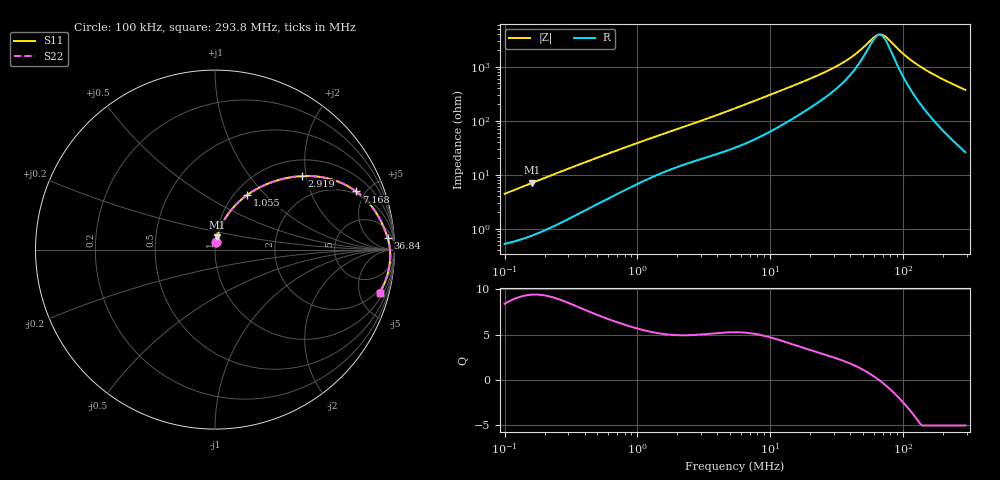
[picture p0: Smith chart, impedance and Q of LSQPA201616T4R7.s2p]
! LSQPA201616T4R7  S-PARAMETER MODEL  ( General Type )
! Model Generated by TAIYO YUDEN Corporation (http://www.ty-top.com)
! Version 2.0
! TAIYO YUDEN Control No. 100810NF25SB-FKC
! Copyright(c) 2007 TAIYO YUDEN CO.,LTD. All Rights Reserved.
! Product Description (link to TY-COMPAS)
! https://ds.yuden.co.jp/TYCOMPAS/or/detail?pn=LSQPA201616T4R7M&u=M
! Products Name : Inductors
! Characteristics :
!  Inductance : 4.7 uH , SRF(min) : 45 MHz , DC Resistance(max) : 0.481 Ohm
!  Rated Current : Saturation :550 mA , Temp Rise : 530 mA (40 degC)
!  Case Size : 2.0 x 1.6 / 0.079 x 0.063 [mm/inch] , Thickness : 1.6 / 0.063 [mm/inch]
!  (Conditions: Temperature = 25 degC , DC Bias Current/Voltage = 0A / 0V)
! External Node Assignments :
!  1  o---GGG---o  2
! GND o---------o GND
! Frequency Range : 0.1MHz  -  293.796821MHz  [ 402 STEP ]
# MHz S RI R 50
! Freq[MHz].  S11 Real  S11 Imag  S21 Real  S21 Imag  S12 Real  S12 Imag  S22 Real  S22 Imag
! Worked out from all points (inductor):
!   401 points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, 100 kHz to 293.8 MHz, reference 50 ohm
!   read as one part in series: L = 6.94 uH near 104.1 kHz
!   highest Q = 9.41 at 161.5 kHz (marker M1), where L = 6.91 uH
!   self-resonance near 65.8 MHz
!   S11 on the Smith chart (normalised r, x): 100 kHz: 1.01, +0.09; 1.055 MHz: 1.14, +0.80; 2.919 MHz: 1.38, +1.90; 7.168 MHz: 1.84, +4.31; 36.84 MHz: 12, +23; 293.8 MHz: 1.52, -7.39
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0.1  0.00706 0.0432  0.9929 -0.0432  0.9929 -0.0432  0.00706 0.0432
0.161467  0.0122 0.0687  0.9878 -0.0687  0.9878 -0.0687  0.0122 0.0687
0.380976  0.0431 0.1493  0.9569 -0.1493  0.9569 -0.1493  0.0431 0.1493
0.653117  0.0952 0.2267  0.9048 -0.2267  0.9048 -0.2267  0.0952 0.2267
1.054566  0.1798 0.3047  0.8202 -0.3047  0.8202 -0.3047  0.1798 0.3047
1.451429  0.2594 0.3517  0.7406 -0.3517  0.7406 -0.3517  0.2594 0.3517
2.919106  0.486 0.4097  0.514 -0.4097  0.514 -0.4097  0.486 0.4097
3.938235  0.5957 0.4034  0.4043 -0.4034  0.4043 -0.4034  0.5957 0.4034
5.420303  0.7063 0.3703  0.2937 -0.3703  0.2937 -0.3703  0.7063 0.3703
7.168119  0.7868 0.3237  0.2132 -0.3237  0.2132 -0.3237  0.7868 0.3237
11.57412  0.8792 0.2319  0.1208 -0.2319  0.1208 -0.2319  0.8792 0.2319
20.65007  0.9344 0.1374  0.0656 -0.1374  0.0656 -0.1374  0.9344 0.1374
28.42126  0.9515 0.0959  0.0485 -0.0959  0.0485 -0.0959  0.9515 0.0959
36.84299  0.9618 0.0655  0.0382 -0.0655  0.0382 -0.0655  0.9618 0.0655
44.98379  0.9679 0.043  0.0321 -0.043  0.0321 -0.043  0.9679 0.043
63.16086  0.9746 0.00473  0.0254 -0.00473  0.0254 -0.00473  0.9746 0.00473
69.79087  0.9757 -0.00686  0.0243 0.00686  0.0243 0.00686  0.9757 -0.00686
78.67184  0.9765 -0.0211  0.0235 0.0211  0.0235 0.0211  0.9765 -0.0211
101.9837  0.9759 -0.0539  0.0241 0.0539  0.0241 0.0539  0.9759 -0.0539
132.2033  0.9717 -0.0905  0.0283 0.0905  0.0283 0.0905  0.9717 -0.0905
193.1855  0.9562 -0.1541  0.0438 0.1541  0.0438 0.1541  0.9562 -0.1541
293.7968  0.9174 -0.2424  0.0826 0.2424  0.0826 0.2424  0.9174 -0.2424
